(* Logix 5000 AddOnInstructionDefinition export Banner_QS18E_Param_v4; software revision 33.00; part 3 of 3 *)
(* tags used below, declared in another part *)
   QS18E : Banner_QS18E_v4;
   Port_Data : Banner_IOL_Port_v4;
   Port : DINT;
   Local_Control : DINT;
   Command_Being_Processed : BOOL;
   Update_Archive : BOOL;
   Index_Write_Inprocess : INT;
   Inprocess_Index : DINT;
(* Banner_QS18E_Param_v4, continued *)

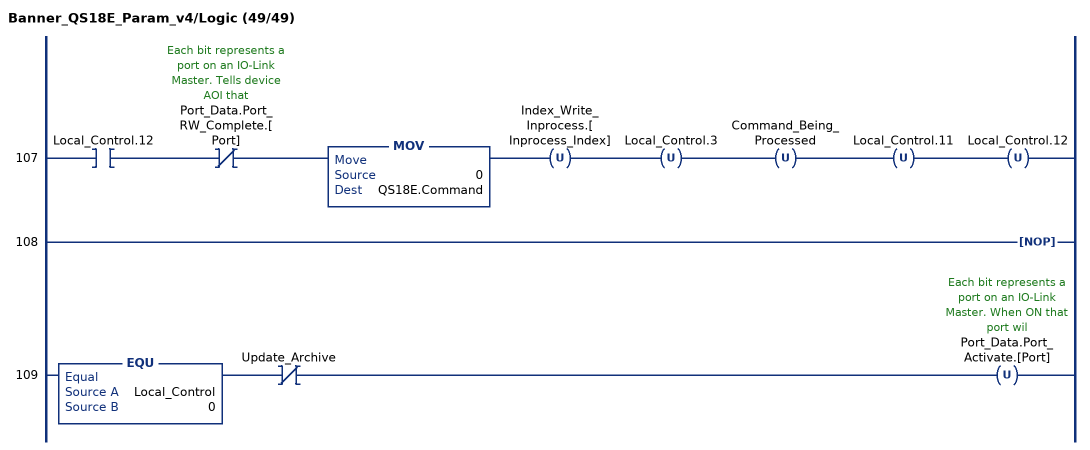
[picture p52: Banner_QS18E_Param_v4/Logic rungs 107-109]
   107: XIC(Local_Control.12)XIO(Port_Data.Port_RW_Complete.[Port])MOV(0,QS18E.Command)OTU(Index_Write_Inprocess.[Inprocess_Index])OTU(Local_Control.3)OTU(Command_Being_Processed)OTU(Local_Control.11)OTU(Local_Control.12);
   108: NOP();
   109: EQU(Local_Control,0)XIO(Update_Archive)OTU(Port_Data.Port_Activate.[Port]);
END_ROUTINE
END_ADD_ON_INSTRUCTION
